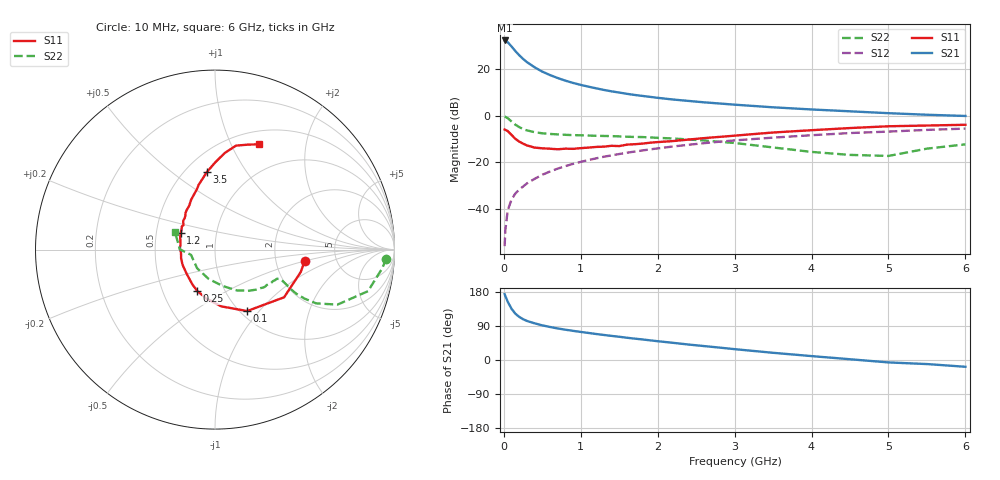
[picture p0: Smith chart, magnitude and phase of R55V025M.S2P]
! SIEMENS Small Signal Semiconductors
! BFR183
! Si NPN RF Bipolar Junction Transistor in SOT23
! VCE = 5 V  IC = 25 mA
! Common Emitter S-Parameters:  May  1996
# GHz  S  MA  R  50
!  f  S11  S21  S12  S22
! GHz  MAG  ANG  MAG  ANG  MAG  ANG  MAG  ANG
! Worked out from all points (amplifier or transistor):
!   36 points, 10 MHz to 6 GHz, reference 50 ohm
!   highest |S21| = 32.2 dB at 10 MHz (marker M1)
!   |S21| within 3 dB of that: start of sweep to 110.7 MHz
!   unconditionally stable (mu >= 1): 526.6 MHz to 2.402 GHz
!   at 250 MHz: K = 0.84, MSG = 27.3 dB, |S12| = -30.4 dB
!   at 1.4 GHz: K = 1.04, MAG = 12.5 dB, |S12| = -17.0 dB
!   at 6 GHz: K = 0.90, MSG = 2.7 dB, |S12| = -5.6 dB
!   S11 on the Smith chart (normalised r, x): 10 MHz: 2.93, -0.50; 100 MHz: 1.08, -0.87; 250 MHz: 0.74, -0.37; 1.2 GHz: 0.67, +0.13; 3.5 GHz: 0.63, +0.68; 6 GHz: 0.65, +1.28
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0.01  0.5032 -7.3  40.64 174.0  0.0016 86.6  0.955 -3.0
0.02  0.494 -14.6  40.17 168.5  0.0036 87.5  0.9376 -6.4
0.05  0.4678 -34.6  37.28 154.0  0.0093 76.8  0.8834 -15.2
0.1  0.3863 -62.4  30.22 135.2  0.016 72.7  0.7479 -24.2
0.15  0.3181 -83.7  24.02 122.1  0.0215 69.0  0.6381 -28.0
0.2  0.2777 -99.7  19.63 113.8  0.026 69.6  0.5664 -28.7
0.25  0.2507 -113.3  16.35 107.7  0.0303 70.0  0.5152 -28.5
0.3  0.2299 -123.7  13.98 103.1  0.0353 71.5  0.4823 -27.7
0.4  0.2063 -141.1  10.82 96.8  0.0443 72.2  0.4417 -26.1
0.5  0.1994 -155.1  8.735 91.4  0.0541 72.9  0.418 -25.0
0.6  0.1954 -164.9  7.376 87.1  0.0635 72.6  0.4048 -24.7
0.7  0.1901 -175.2  6.378 83.3  0.0732 72.4  0.3954 -24.5
0.8  0.1959 178.0  5.599 80.0  0.0829 71.8  0.3877 -24.9
0.9  0.1941 171.9  5.006 76.9  0.0927 71.4  0.3821 -25.1
1.1  0.2067 159.7  4.163 71.4  0.1118 70.0  0.3739 -27.3
1.2  0.2134 153.5  3.839 68.6  0.1216 69.3  0.3693 -28.1
1.6  0.2389 137.9  2.924 58.7  0.1603 65.4  0.3526 -33.4
2.2  0.2849 120.1  2.209 45.3  0.2182 58.8  0.3234 -43.4
3.5  0.4345 96.0  1.505 19.0  0.3375 42.5  0.2079 -77.8
4.5  0.5412 84.2  1.235 2.0  0.4231 29.8  0.144 -133.9
5.5  0.6128 72.6  1.043 -10.7  0.494 18.2  0.1961 179.5
6  0.636 67.3  0.982 -17.9  0.527 10.7  0.2421 156.6
